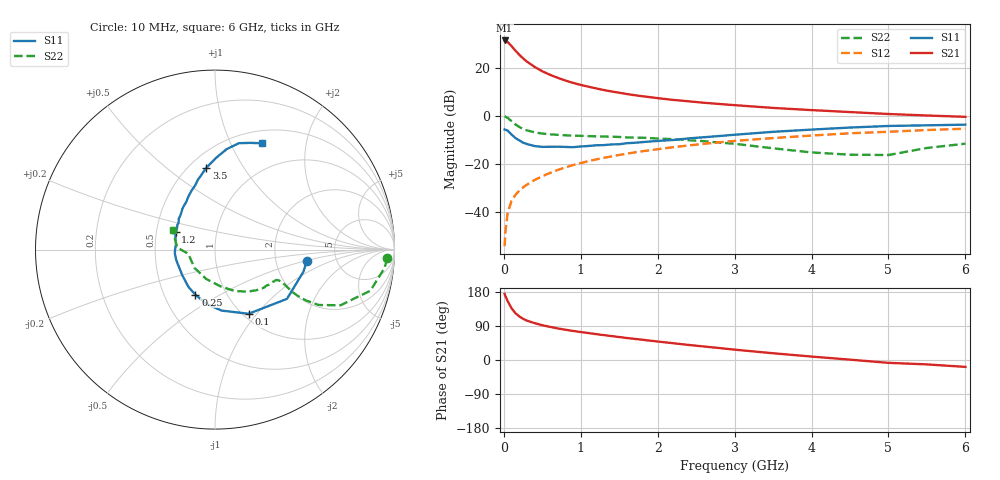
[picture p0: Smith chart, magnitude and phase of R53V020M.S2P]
! SIEMENS Small Signal Semiconductors
! BFR183
! Si NPN RF Bipolar Junction Transistor in SOT23
! VCE = 3 V  IC = 20 mA
! Common Emitter S-Parameters:  May  1996
# GHz  S  MA  R  50
!  f  S11  S21  S12  S22
! GHz  MAG  ANG  MAG  ANG  MAG  ANG  MAG  ANG
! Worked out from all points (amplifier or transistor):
!   36 points, 10 MHz to 6 GHz, reference 50 ohm
!   highest |S21| = 31.3 dB at 10 MHz (marker M1)
!   |S21| within 3 dB of that: start of sweep to 117.5 MHz
!   unconditionally stable (mu >= 1): 529.8 MHz to 2.359 GHz
!   at 250 MHz: K = 0.81, MSG = 26.9 dB, |S12| = -29.9 dB
!   at 1.4 GHz: K = 1.04, MAG = 12.2 dB, |S12| = -17.0 dB
!   at 6 GHz: K = 0.90, MSG = 2.5 dB, |S12| = -5.5 dB
!   S11 on the Smith chart (normalised r, x): 10 MHz: 3.02, -0.53; 100 MHz: 1.06, -0.91; 250 MHz: 0.72, -0.39; 1.2 GHz: 0.63, +0.13; 3.5 GHz: 0.60, +0.70; 6 GHz: 0.65, +1.32
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0.01  0.5146 -7.2  36.77 174.6  0.0019 85.6  0.9622 -2.9
0.02  0.5079 -14.0  36.52 169.2  0.0038 74.6  0.9492 -6.3
0.05  0.4859 -34.4  34.13 155.2  0.0095 78.6  0.8958 -14.8
0.1  0.4036 -62.3  28.08 136.7  0.0167 71.0  0.7652 -23.9
0.15  0.3419 -83.8  22.61 123.5  0.0221 68.5  0.6556 -28.1
0.2  0.3051 -99.5  18.6 115.2  0.0271 68.2  0.581 -29.2
0.25  0.2735 -113.6  15.55 108.7  0.0319 68.1  0.5275 -29.2
0.3  0.2555 -125.2  13.33 103.9  0.0364 69.0  0.4919 -28.7
0.4  0.2317 -141.6  10.34 97.3  0.0454 70.3  0.4482 -27.2
0.5  0.2229 -154.7  8.375 91.7  0.0545 71.5  0.4215 -26.2
0.6  0.2237 -164.5  7.073 87.4  0.0638 71.5  0.4073 -25.8
0.7  0.2248 -174.6  6.124 83.4  0.0736 71.4  0.3969 -25.8
0.8  0.2222 179.5  5.373 79.9  0.0832 70.9  0.3882 -26.0
0.9  0.2194 171.9  4.804 76.7  0.0932 70.6  0.3822 -26.3
1.1  0.2323 161.1  3.996 71.1  0.1123 69.5  0.3735 -28.3
1.2  0.2405 155.7  3.684 68.2  0.1221 68.7  0.3684 -29.2
1.6  0.2657 139.4  2.808 58.0  0.1607 64.9  0.3513 -34.6
2.2  0.31 121.2  2.123 44.3  0.2191 58.8  0.3223 -44.8
3.5  0.4586 96.0  1.445 17.8  0.3401 42.3  0.208 -81.1
4.5  0.5633 83.4  1.184 0.9  0.4278 29.6  0.1531 -138.6
5.5  0.6267 71.6  1.004 -11.6  0.4999 17.8  0.2115 176.8
6  0.647 66.3  0.942 -18.2  0.5331 10.2  0.2598 155.0
